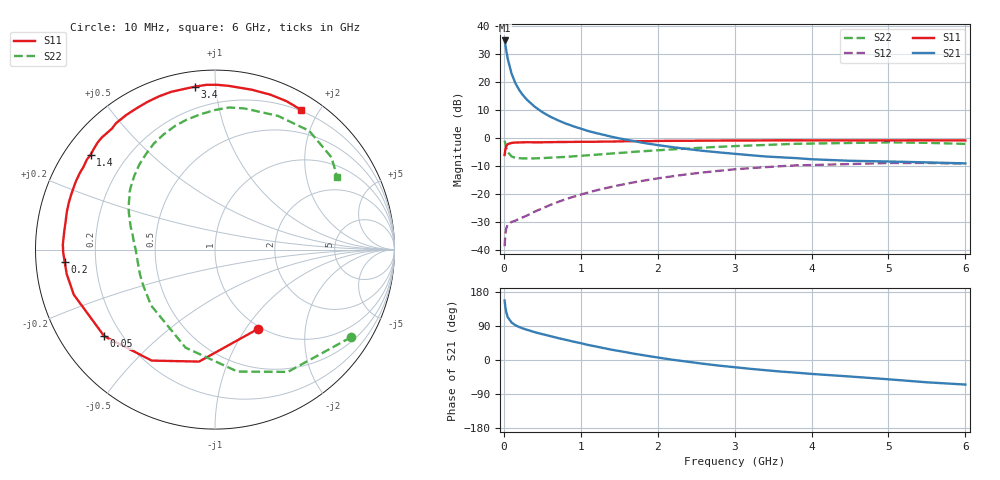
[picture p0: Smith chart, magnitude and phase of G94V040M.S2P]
! SIEMENS Small Signal Semiconductors
! BFG235
! Si NPN RF Bipolar Junction Transistor in SOT223
! VCE = 4 V  IC = 40 mA
! Common Emitter S-Parameters:  July  1994
# GHz  S  MA  R  50
!  f  S11  S21  S12  S22
! GHz  MAG  ANG  MAG  ANG  MAG  ANG  MAG  ANG
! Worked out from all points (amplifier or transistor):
!   40 points, 10 MHz to 6 GHz, reference 50 ohm
!   highest |S21| = 34.9 dB at 10 MHz (marker M1)
!   |S21| within 3 dB of that: start of sweep to 28.28 MHz
!   unconditionally stable (mu >= 1): 506.5 MHz to 1.407 GHz
!   at 200 MHz: K = 0.62, MSG = 23.0 dB, |S12| = -28.7 dB
!   at 1.5 GHz: K = 0.98, MSG = 8.3 dB, |S12| = -16.7 dB
!   at 6 GHz: K = 0.94, MSG = 0.1 dB, |S12| = -9.1 dB
!   S11 on the Smith chart (normalised r, x): 10 MHz: 0.96, -1.14; 50 MHz: 0.14, -0.34; 200 MHz: 0.09, -0.04; 1.4 GHz: 0.08, +0.34; 3.4 GHz: 0.08, +0.88; 6 GHz: 0.19, +1.78
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0.01  0.5026 -61.8  55.38 157.1  0.0119 68.9  0.9023 -32.7
0.02  0.6302 -98.1  46.19 139.6  0.0196 53.8  0.7932 -59.2
0.03  0.7119 -119.7  37.89 127.6  0.0245 44.2  0.6913 -79.5
0.05  0.7834 -142.0  26.3 113.4  0.0286 32.8  0.5704 -106.7
0.1  0.8258 -162.3  14.25 98.9  0.0322 28.1  0.4729 -138.8
0.15  0.8373 -170.6  9.617 91.8  0.0339 30.4  0.4476 -153.1
0.2  0.8404 -175.2  7.221 87.0  0.0366 33.3  0.4407 -161.1
0.25  0.8458 -178.9  5.817 83.1  0.0391 36.8  0.4368 -166.4
0.3  0.8482 178.1  4.863 79.8  0.0418 39.8  0.436 -170.5
0.4  0.846 173.2  3.662 73.6  0.049 44.3  0.4378 -176.0
0.5  0.8467 169.4  2.92 68.2  0.0562 47.5  0.4424 179.9
0.6  0.8517 165.8  2.436 63.3  0.0643 49.3  0.4495 176.3
0.7  0.8556 162.3  2.099 58.1  0.0727 50.8  0.4575 173.1
0.9  0.86 156.6  1.641 48.7  0.09 50.7  0.4749 167.6
1.1  0.8657 150.2  1.341 39.5  0.1081 49.6  0.4972 162.2
1.4  0.872 142.6  1.064 27.2  0.1357 45.9  0.5342 154.2
2.2  0.8983 123.4  0.692 0.5  0.2106 30.6  0.6345 131.6
3.2  0.9111 101.4  0.499 -23.2  0.2924 6.7  0.7408 102.3
3.4  0.9148 97.0  0.473 -26.9  0.3049 1.6  0.7584 96.1
4.5  0.9141 77.1  0.396 -43.6  0.3466 -24.6  0.8235 64.8
5.5  0.9179 64.2  0.371 -58.9  0.3628 -47.0  0.8279 38.4
6  0.9146 58.3  0.356 -64.8  0.3516 -55.2  0.7924 30.9
